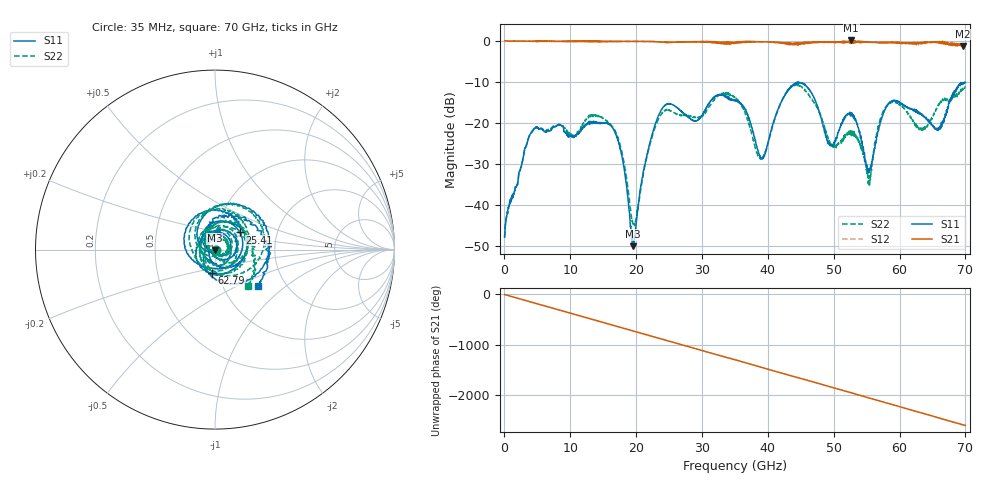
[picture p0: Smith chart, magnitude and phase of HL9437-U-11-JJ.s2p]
! 7/27/2020 10:55:55 AM
! H:\PRODUCTION_DATA\TEMP_S2P.S2P
! CHANNEL.1
! TR.MEASUREMENT
! CORRECTED.DATA
# GHZ S RI R 50.0
! FREQ.GHZ  S11RE  S11IM  S21RE  S21IM  S12RE  S12IM  S22RE  S22IM
!; PortSelection: Port_12
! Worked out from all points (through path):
!   2000 points, 35 MHz to 70 GHz, reference 50 ohm
!   highest |S21| = 0.06 dB at 52.64 GHz (marker M1); lowest = -1.3 dB at 69.58 GHz (marker M2)
!   group delay of S21, straight-line fit = 104 ps
!   lowest |S11| = -50.0 dB at 19.57 GHz (marker M3), VSWR 1.01, Z = 49.9 - j0.304 ohm
!   |S11| at or under -10 dB: start of sweep to end of sweep
!   |S22| runs from -47.9 to -10.6 dB; largest |S21 - S12| = 0.1
!   S11 on the Smith chart (normalised r, x): 35 MHz: 1.01, -0.00; 25.41 GHz: 1.29, +0.25; 62.79 GHz: 0.94, -0.25; 70 GHz: 1.45, -0.65
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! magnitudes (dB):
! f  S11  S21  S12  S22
! 35 MHz  -47.8  0.0  0.0  -47.9
! 4.235 GHz  -22.2  -0.1  -0.1  -22.0
! 11.72 GHz  -21.6  -0.2  -0.1  -20.9
! 16.77 GHz  -22.1  -0.2  -0.2  -21.7
! 18.02 GHz  -29.6  -0.2  -0.2  -28.4
! 19.57 GHz  -50.0  -0.2  -0.2  -44.6
! 21.28 GHz  -30.4  -0.2  -0.2  -30.9
! 23.38 GHz  -18.3  -0.3  -0.2  -19.2
! 25.41 GHz  -15.5  -0.4  -0.3  -17.2
! 28.98 GHz  -19.5  -0.3  -0.3  -18.6
! 35.03 GHz  -14.5  -0.4  -0.4  -13.9
! 38.95 GHz  -28.6  -0.2  -0.3  -28.7
! 43.23 GHz  -11.7  -0.6  -1.0  -11.6
! 46.69 GHz  -12.8  -0.5  -0.3  -14.2
! 49.63 GHz  -25.3  -0.4  -0.3  -25.4
! 52.64 GHz  -17.8  0.1  -0.5  -22.6
! 55.34 GHz  -32.1  -0.4  -0.4  -32.8
! 58.34 GHz  -15.3  -0.5  -0.4  -15.3
! 62.79 GHz  -17.6  -0.7  -0.5  -21.3
! 65.97 GHz  -21.6  -0.2  -0.6  -15.7
! 69.58 GHz  -10.3  -1.3  -1.0  -11.6
! 70 GHz  -10.2  -1.0  -1.1  -11.3
